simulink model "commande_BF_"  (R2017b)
settings: Solver=ode1  StartTime=0.0  StopTime=150  FixedStep=0.001  RelTol=1e-3
undefined symbols (not defined in the file or in its folder): Advantech, PCI
libraries: sldrtlib x11

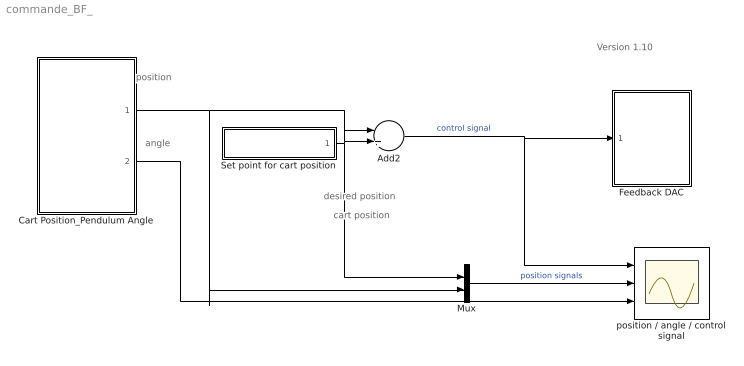
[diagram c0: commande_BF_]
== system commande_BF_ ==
  note: position
  note: angle
  note: desired position
  note: cart position
  note: Version 1.10
  Add2 : Sum  Inputs=-+
  Cart Position_Pendulum Angle : Subsystem  mask(Feedback Encoder Block){st=0.001, of1=0, of2=-1024}
      mask prompts: st "Sample Time"; of1 "Channel 1 Offset"; of2 "Channel 2 Offset"
      mask help: Special block to use with the Feedback experiments to read encoder channels using the digital I/O lines
  Feedback DAC : Subsystem  mask(DAC Unit for Feedback Experiments){st=0.001, ch=1}
      mask prompts: st "Sample Time"; ch "Output Channel"
      mask help: Digital to Analog Output for Feedback Experiments using Advantech PCI1711 I/O board
  Mux : Mux  Inputs=2
  Set point for cart position : Subsystem
  position / angle / control signal : Scope  NumInputPorts=3
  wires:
  Set point for cart position/1(desired position) -> Add2/2, Mux/1
  Cart Position_Pendulum Angle/1(Channel 1) -> Add2/1, Mux/2
  Add2/1 -> position / angle / control signal/1, Feedback DAC/1(In1)  "control signal"
  Cart Position_Pendulum Angle/2(Channel 2) -> position / angle / control signal/3
  Mux/1 -> position / angle / control signal/2  "position signals"

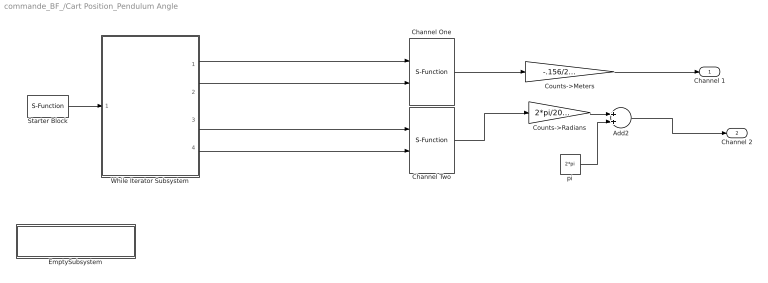
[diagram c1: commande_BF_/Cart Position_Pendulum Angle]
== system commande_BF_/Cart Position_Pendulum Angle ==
  Add2 : Sum
  Channel One : S-Function  FunctionName=Converter  Parameters=of1,st  SFunctionDeploymentMode=off  EnableBusSupport=off
  Channel Two : S-Function  FunctionName=Converter  Parameters=of2,st  SFunctionDeploymentMode=off  EnableBusSupport=off
  Counts->Meters : Gain  Gain=-.156/2048
  Counts->Radians : Gain  Gain=2*pi/2048
  EmptySubsystem : Subsystem
  Starter Block : S-Function  FunctionName=Starter  Parameters=sample_time  SFunctionDeploymentMode=off  EnableBusSupport=off  mask{sample_time=st}
      mask prompts: sample_time "Sample Time:"
  While Iterator Subsystem : Subsystem  TreatAsAtomicUnit=on
  pi : Constant  Value=2*pi
  Channel 1 : Outport
  Channel 2 : Outport  Port=2
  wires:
  Add2/1 -> Channel 2/1
  Channel Two/1 -> Counts->Radians/1
  pi/1 -> Add2/2
  Counts->Radians/1 -> Add2/1
  Counts->Meters/1 -> Channel 1/1
  Starter Block/1 -> While Iterator Subsystem/1(In1)
  While Iterator Subsystem/1(Out1) -> Channel One/1
  While Iterator Subsystem/2(Out3) -> Channel One/2
  While Iterator Subsystem/3(Out2) -> Channel Two/1
  While Iterator Subsystem/4(Out4) -> Channel Two/2
  Channel One/1 -> Counts->Meters/1

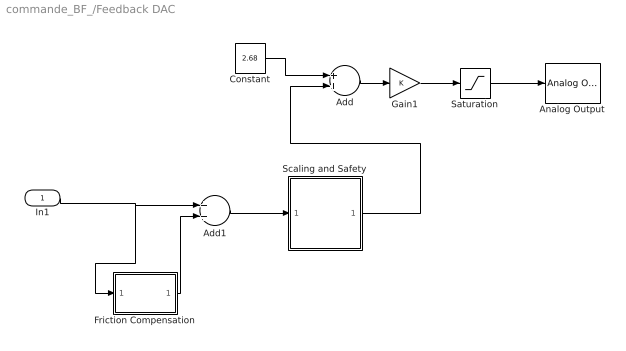
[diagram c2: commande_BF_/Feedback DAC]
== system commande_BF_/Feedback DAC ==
  In1 : Inport
  Add : Sum
  Add1 : Sum
  Analog Output : sldrtlib/Analog Output  SampleTime=st  MaxMissedTicks=10  ShowMissedTicks=off  YieldWhenWaiting=off  DrvName=Advantech/PCI-1711  DrvAddress=4294967295  DrvOptions=zeros(1,0)  Channels=ch  RangeMode=1  VoltRange=2  InitialValue=2.5  FinalValue=2.5
  Constant : Constant  Value=2.68
  Friction Compensation : Subsystem  mask(linear){frictionCompNeg=.1, frictionCompPos=.1}
      mask prompts: frictionCompNeg "Friction Compensation Magnitude in Negative Direction"; frictionCompPos "Friction Compensation Magnitude in Positive Direction"
  Gain1 : Gain
  Saturation : Saturate  UpperLimit=5.0  LowerLimit=0
  Scaling and Safety : Subsystem
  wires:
  Scaling and Safety/1(Out1) -> Add/2
  Gain1/1 -> Saturation/1
  Add/1 -> Gain1/1
  Saturation/1 -> Analog Output/1
  Constant/1 -> Add/1
  Friction Compensation/1(Out1) -> Add1/2
  In1/1 -> Friction Compensation/1(In1), Add1/1
  Add1/1 -> Scaling and Safety/1(In1)

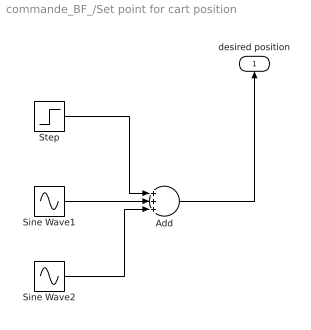
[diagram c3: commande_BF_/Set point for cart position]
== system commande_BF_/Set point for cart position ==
  Add : Sum  Inputs=+++
  Sine Wave1 : Sin  Amplitude=0  Frequency=20  SampleTime=0
  Sine Wave2 : Sin  Amplitude=0  Frequency=7  SampleTime=0
  Step : Step  After=0.2  SampleTime=0
  desired position : Outport
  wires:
  Step/1 -> Add/1
  Add/1 -> desired position/1
  Sine Wave1/1 -> Add/2
  Sine Wave2/1 -> Add/3

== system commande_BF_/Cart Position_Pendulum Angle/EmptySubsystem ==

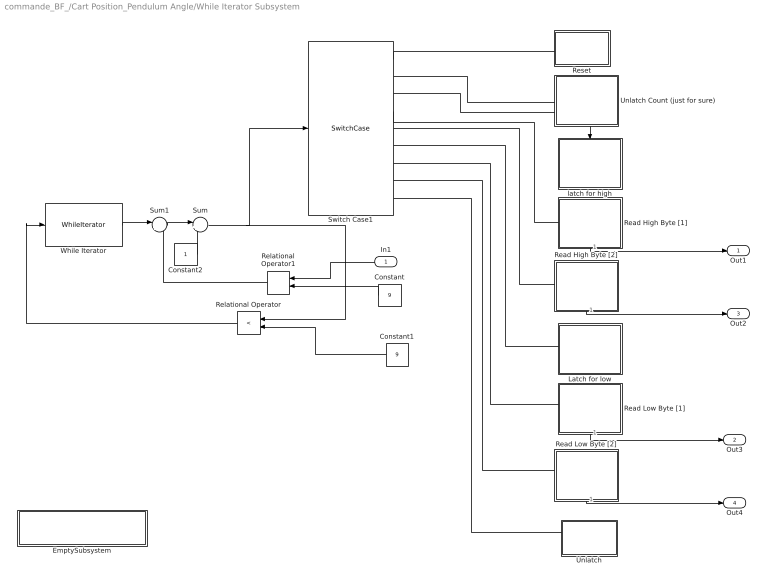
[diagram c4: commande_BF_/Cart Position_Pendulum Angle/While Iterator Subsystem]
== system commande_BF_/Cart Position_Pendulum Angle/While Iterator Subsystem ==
  In1 : Inport
  Constant : Constant  Value=9
  Constant1 : Constant  Value=9
  Constant2 : Constant
  EmptySubsystem : Subsystem
  Latch for low : Subsystem  TreatAsAtomicUnit=on
  Read High Byte [1] : Subsystem  TreatAsAtomicUnit=on
  Read High Byte [2] : Subsystem  TreatAsAtomicUnit=on
  Read Low Byte [1] : Subsystem  TreatAsAtomicUnit=on
  Read Low Byte [2] : Subsystem  TreatAsAtomicUnit=on
  Relational Operator : RelationalOperator  Operator=<  OutDataTypeStr=boolean
  Relational Operator1 : RelationalOperator  Operator===  OutDataTypeStr=boolean
  Reset : Subsystem  TreatAsAtomicUnit=on
  Sum : Sum  Inputs=|++
  Sum1 : Sum  Inputs=|+-
  Switch Case1 : SwitchCase  CaseConditions={1,2,3,4,5,6,7,8,9}  ShowDefaultCase=off
  Unlatch : Subsystem  TreatAsAtomicUnit=on
  "Unlatch Count (just for sure) " : Subsystem  TreatAsAtomicUnit=on
  While Iterator : WhileIterator  MaxIters=9  WhileBlockType=do-while  ResetStates=reset  ShowIterationPort=on  OutputDataType=int8
  latch for high : Subsystem  TreatAsAtomicUnit=on
  Out1 : Outport
  Out3 : Outport  Port=2
  Out2 : Outport  Port=3
  Out4 : Outport  Port=4
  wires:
  Relational Operator/1 -> While Iterator/1
  In1/1 -> Relational Operator1/1
  Constant/1 -> Relational Operator1/2
  Relational Operator1/1 -> Sum1/2
  While Iterator/1 -> Sum1/1
  Switch Case1/1 -> Reset/Action
  Switch Case1/2 -> "Unlatch Count (just for sure) "/Action
  Constant1/1 -> Relational Operator/2
  Read High Byte [1]/1(Out2) -> Out1/1
  Read High Byte [2]/1(Out2) -> Out2/1
  Read Low Byte [1]/1(Out2) -> Out3/1
  Read Low Byte [2]/1(Out2) -> Out4/1
  Sum1/1 -> Sum/1
  Sum/1 -> Switch Case1/1, Relational Operator/1
  Constant2/1 -> Sum/2
  Switch Case1/3 -> latch for high/Action
  Switch Case1/4 -> Read High Byte [1]/Action
  Switch Case1/5 -> Read High Byte [2]/Action
  Switch Case1/6 -> Latch for low/Action
  Switch Case1/7 -> Read Low Byte [1]/Action
  Switch Case1/8 -> Read Low Byte [2]/Action
  Switch Case1/9 -> Unlatch/Action

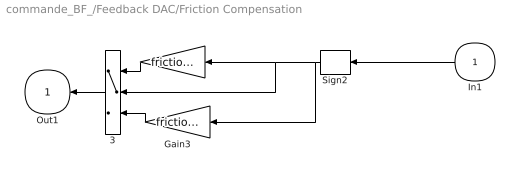
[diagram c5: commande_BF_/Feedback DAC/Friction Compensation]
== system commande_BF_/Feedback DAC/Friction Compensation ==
  In1 : Inport
  " " : Gain  Gain=frictionCompPos
  3 : Switch
  Gain3 : Gain  Gain=frictionCompNeg
  Sign2 : Signum  Tag=T
  Out1 : Outport  InitialOutput=0
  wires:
  In1/1 -> Sign2/1
  " "/1 -> 3/1
  Gain3/1 -> 3/3
  Sign2/1 -> Gain3/1, " "/1, 3/2
  3/1 -> Out1/1

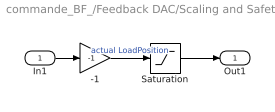
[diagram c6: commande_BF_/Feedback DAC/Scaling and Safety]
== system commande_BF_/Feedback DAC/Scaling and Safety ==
  In1 : Inport
  -1 : Gain  Gain=-1
  Saturation : Saturate  UpperLimit=2.5  LowerLimit=-2.5
  Out1 : Outport
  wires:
  Saturation/1 -> Out1/1
  In1/1 -> -1/1
  -1/1 -> Saturation/1  "actual LoadPosition"

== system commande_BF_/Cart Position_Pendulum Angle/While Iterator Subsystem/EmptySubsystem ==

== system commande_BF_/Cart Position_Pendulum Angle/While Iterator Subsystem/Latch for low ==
  Action Port : ActionPort  ActionType=case
  Constant : Constant  Value=6  OutDataTypeStr=double
  Digital Output : sldrtlib/Digital Output  SampleTime=-1  MaxMissedTicks=10  ShowMissedTicks=off  YieldWhenWaiting=off  DrvName=Advantech/PCI-1711  DrvAddress=4294967295  DrvOptions=zeros(1,0)  Channels=1  BitMode=2  InitialValue=0  FinalValue=0
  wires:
  Constant/1 -> Digital Output/1

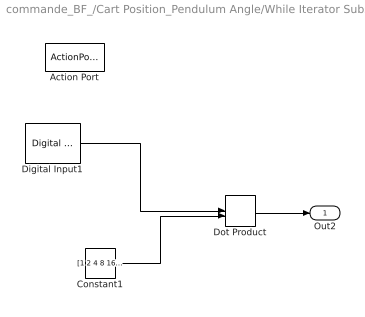
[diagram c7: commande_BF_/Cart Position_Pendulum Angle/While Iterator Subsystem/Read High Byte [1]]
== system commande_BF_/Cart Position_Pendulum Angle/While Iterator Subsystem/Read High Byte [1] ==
  Action Port : ActionPort  ActionType=case
  Constant1 : Constant  Value=[1 2 4 8 16 32 64 128]
  Digital Input1 : sldrtlib/Digital Input  SampleTime=-1  MaxMissedTicks=10  ShowMissedTicks=off  YieldWhenWaiting=off  DrvName=Advantech/PCI-1711  DrvAddress=4294967295  DrvOptions=zeros(1,0)  Channels=[1,2,3,4,5,6,7,8]  BitMode=1  DataType=1
  Dot Product : DotProduct
  Out2 : Outport
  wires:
  Dot Product/1 -> Out2/1
  Constant1/1 -> Dot Product/2
  Digital Input1/1 -> Dot Product/1

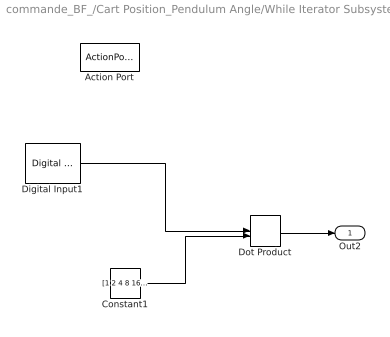
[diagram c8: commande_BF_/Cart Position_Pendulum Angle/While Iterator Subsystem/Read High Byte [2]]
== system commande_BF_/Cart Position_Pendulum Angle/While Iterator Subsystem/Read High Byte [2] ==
  Action Port : ActionPort  ActionType=case
  Constant1 : Constant  Value=[1 2 4 8 16 32 64 128]
  Digital Input1 : sldrtlib/Digital Input  SampleTime=-1  MaxMissedTicks=10  ShowMissedTicks=off  YieldWhenWaiting=off  DrvName=Advantech/PCI-1711  DrvAddress=4294967295  DrvOptions=zeros(1,0)  Channels=[9:16]  BitMode=1  DataType=1
  Dot Product : DotProduct
  Out2 : Outport
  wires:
  Digital Input1/1 -> Dot Product/1
  Constant1/1 -> Dot Product/2
  Dot Product/1 -> Out2/1

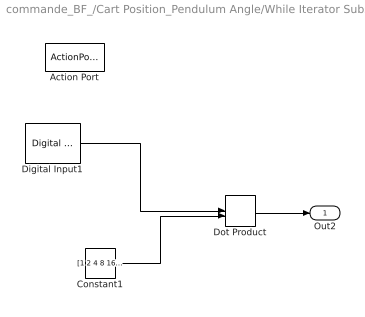
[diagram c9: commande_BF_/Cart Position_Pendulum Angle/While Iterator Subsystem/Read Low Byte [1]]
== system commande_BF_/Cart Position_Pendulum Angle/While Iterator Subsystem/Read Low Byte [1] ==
  Action Port : ActionPort  ActionType=case
  Constant1 : Constant  Value=[1 2 4 8 16 32 64 128]
  Digital Input1 : sldrtlib/Digital Input  SampleTime=-1  MaxMissedTicks=10  ShowMissedTicks=off  YieldWhenWaiting=off  DrvName=Advantech/PCI-1711  DrvAddress=4294967295  DrvOptions=zeros(1,0)  Channels=[1:8]  BitMode=1  DataType=1
  Dot Product : DotProduct
  Out2 : Outport
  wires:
  Digital Input1/1 -> Dot Product/1
  Constant1/1 -> Dot Product/2
  Dot Product/1 -> Out2/1

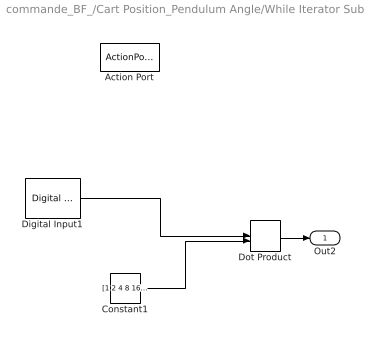
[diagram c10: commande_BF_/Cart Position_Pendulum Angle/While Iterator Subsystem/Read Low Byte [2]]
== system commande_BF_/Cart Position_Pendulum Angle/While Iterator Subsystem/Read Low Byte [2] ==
  Action Port : ActionPort  ActionType=case
  Constant1 : Constant  Value=[1 2 4 8 16 32 64 128]
  Digital Input1 : sldrtlib/Digital Input  SampleTime=-1  MaxMissedTicks=10  ShowMissedTicks=off  YieldWhenWaiting=off  DrvName=Advantech/PCI-1711  DrvAddress=4294967295  DrvOptions=zeros(1,0)  Channels=[9:16]  BitMode=1  DataType=1
  Dot Product : DotProduct
  Out2 : Outport
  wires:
  Constant1/1 -> Dot Product/2
  Digital Input1/1 -> Dot Product/1
  Dot Product/1 -> Out2/1

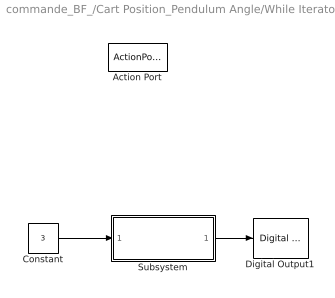
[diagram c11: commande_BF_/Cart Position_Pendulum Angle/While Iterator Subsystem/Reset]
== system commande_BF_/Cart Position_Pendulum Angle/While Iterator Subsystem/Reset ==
  Action Port : ActionPort  ActionType=case
  Constant : Constant  Value=3  OutDataTypeStr=double
  Digital Output1 : sldrtlib/Digital Output  SampleTime=-1  MaxMissedTicks=10  ShowMissedTicks=off  YieldWhenWaiting=off  DrvName=Advantech/PCI-1711  DrvAddress=4294967295  DrvOptions=zeros(1,0)  Channels=1  BitMode=2  InitialValue=0  FinalValue=0
  Subsystem : Subsystem
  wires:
  Constant/1 -> Subsystem/1(In1)
  Subsystem/1(Out1) -> Digital Output1/1

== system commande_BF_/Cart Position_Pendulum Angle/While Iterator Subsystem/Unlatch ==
  Action Port : ActionPort  ActionType=case
  Constant : Constant  Value=7  OutDataTypeStr=double
  Digital Output1 : sldrtlib/Digital Output  SampleTime=-1  MaxMissedTicks=10  ShowMissedTicks=off  YieldWhenWaiting=off  DrvName=Advantech/PCI-1711  DrvAddress=4294967295  DrvOptions=zeros(1,0)  Channels=1  BitMode=2  InitialValue=0  FinalValue=0
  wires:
  Constant/1 -> Digital Output1/1

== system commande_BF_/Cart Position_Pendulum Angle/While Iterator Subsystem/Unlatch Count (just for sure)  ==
  Action Port : ActionPort  ActionType=case
  Constant : Constant  Value=7  OutDataTypeStr=double
  Digital Output : sldrtlib/Digital Output  SampleTime=-1  MaxMissedTicks=10  ShowMissedTicks=off  YieldWhenWaiting=off  DrvName=Advantech/PCI-1711  DrvAddress=4294967295  DrvOptions=zeros(1,0)  Channels=1  BitMode=2  InitialValue=0  FinalValue=0
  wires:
  Constant/1 -> Digital Output/1

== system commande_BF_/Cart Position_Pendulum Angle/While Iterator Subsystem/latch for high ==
  Action Port : ActionPort  ActionType=case
  Constant : Constant  Value=4  OutDataTypeStr=double
  Digital Output : sldrtlib/Digital Output  SampleTime=-1  MaxMissedTicks=10  ShowMissedTicks=off  YieldWhenWaiting=off  DrvName=Advantech/PCI-1711  DrvAddress=4294967295  DrvOptions=zeros(1,0)  Channels=1  BitMode=2  InitialValue=0  FinalValue=0
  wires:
  Constant/1 -> Digital Output/1

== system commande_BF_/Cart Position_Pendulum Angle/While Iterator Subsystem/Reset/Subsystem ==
  In1 : Inport
  Constant1 : Constant  Value=7  OutDataTypeStr=double
  Digital Output : sldrtlib/Digital Output  SampleTime=-1  MaxMissedTicks=10  ShowMissedTicks=off  YieldWhenWaiting=off  DrvName=Advantech/PCI-1711  DrvAddress=4294967295  DrvOptions=zeros(1,0)  Channels=[1 2 3]  BitMode=2  InitialValue=0  FinalValue=0
  Out1 : Outport
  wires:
  Constant1/1 -> Out1/1
  In1/1 -> Digital Output/1
